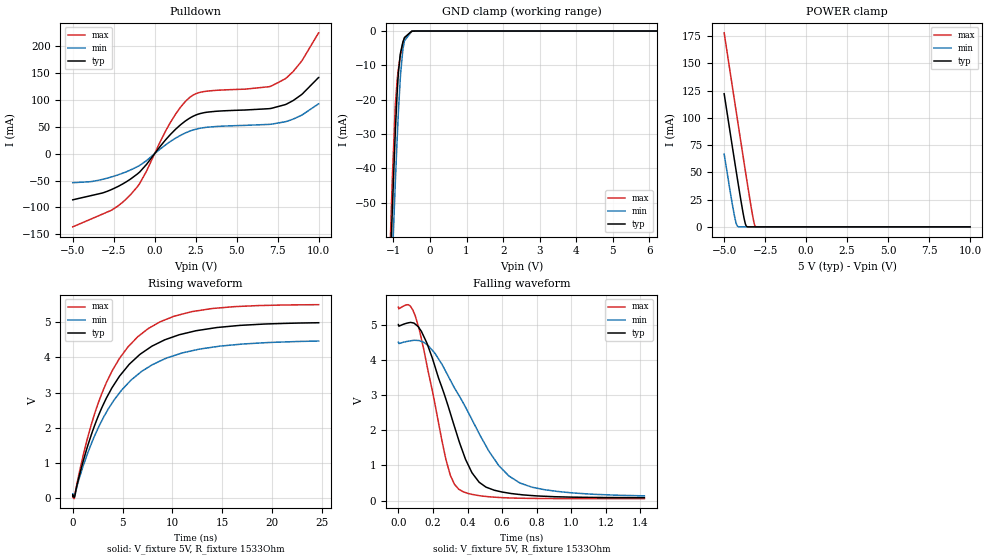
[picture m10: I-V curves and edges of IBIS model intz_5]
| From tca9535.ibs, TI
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|   intz_5 Model
[Model]   intz_5
Model_type   Open_sink
Polarity   Non-Inverting
Vmeas = 2.5
Vref = 5
Cref = 100pF
Rref = 1533
|   typ   min   max
|   (nom PVT)   (fast PVT)   (slow PVT)
C_comp   3.209e-12   3.204e-12   3.540e-12
| Where nom  PVT is Nominal Process, 5V, 27C
|   Fast PVT is Strong Process,  5.5V, -40C
|   Slow PVT is Weak Process,   4.5V, 100C
[Voltage Range]   5   4.5   5.5
|Junction Temperature
[Temperature Range]   27   100   -40
[Pullup Reference]   5   4.5   5.5
[Pulldown Reference]   0   0   0
[Power Clamp Reference]   5   4.5   5.5
[GND Clamp Reference]   0   0   0
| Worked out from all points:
|   slope of the pulldown table from 0 to 0.75 V, typ, clamps not added: 26.3 ohm
|   GND clamp passes 1 mA (typ) near -0.60 V on its own axis
|   POWER clamp passes 1 mA (typ) near -3.66 V on its own axis
|   falling waveform, V_fixture 5V, R_fixture 1533Ohm: 20-80 % time 201ps typ, 301ps min, 135ps max; typ from 5 V to 0.084 V
|   rising waveform, V_fixture 5V, R_fixture 1533Ohm: 20-80 % time 5.37ns typ, 5.74ns min, 4.93ns max; typ from 0.078 V to 4.98 V
[Pulldown]
|   Voltage   I(typ)   I(min)   I(max)
-5V       -85.83mA   -54.02mA   -136.1mA
-2.635V   -66.76mA   -43.31mA   -105.2mA
-1.486V   -47.45mA   -30.49mA   -76.69mA
-913.5mV  -33.98mA   -21.71mA   -55.33mA
967.5mV   36.03mA    22.95mA    58.62mA
2.117V    65.81mA    41.68mA    104.2mA
3.1V      76.74mA    48.82mA    116mA
7.101V    84.21mA    54.81mA    125.6mA
7.958V    91.23mA    59.35mA    139.2mA
8.447V    98.85mA    64.3mA     152.9mA
9.004V    111.1mA    72.36mA    174.1mA
10V       141.8mA    92.78mA    224.8mA
[GND Clamp]
|   Voltage   I(typ)   I(min)   I(max)
-5V       -1.737A    -1.579A    -1.998A
-1.085V   -68.6mA    -82.69mA   -60.63mA
-1.034V   -52.99mA   -67.79mA   -44mA
-1.03V    -51.64mA   -66.48mA   -42.61mA
-946.5mV  -28.53mA   -43.34mA   -21.14mA
-900.5mV  -18.27mA   -31.74mA   -14.42mA
-875mV    -13.78mA   -25.83mA   -11.89mA
-815mV    -6.977mA   -14.08mA   -7.383mA
-743mV    -3.229mA   -5.373mA   -3.548mA
-699mV    -1.904mA   -2.808mA   -1.974mA
-500mV    -56.39uA   -109.9uA   -29.75uA
10V       0A         0A         0A
[POWER Clamp]
|   Voltage   I(typ)   I(min)   I(max)
-5V       122.2mA    66.83mA    178.2mA
-4.519V   75.31mA    22.22mA    130.6mA
-4.343V   58.41mA    7.966mA    113.4mA
-4.235V   48.11mA    1.854mA    102.8mA
-4.15V    40.09mA    219.4uA    94.43mA
-3.865V   14.26mA    47.82nA    66.64mA
-3.71V    2.889mA    13.4nA     51.65mA
-3.61V    172.9uA    12.3nA     42.06mA
-3.272V   0A         0A         10.96mA
-3.163V   0A         0A         2.802mA
-3.091V   0A         0A         279.9uA
10V       0A         0A         0A
[Ramp]
R_load = 1533
|   typ   min   max
dV/dt_r   2.95311/5.42004e-09   2.63427/5.89243e-09   3.26857/4.94307e-09
dV/dt_f   2.95311/2.01074e-10   2.63427/3.0361e-10   3.26857/1.35007e-10
[Falling Waveform]
V_fixture = 5V
V_fixture_min = 4.5V
V_fixture_max = 5.5V
R_fixture = 1533Ohm
|   Time   V(typ)   V(min)   V(max)
0s        5V         4.5V       5.5V
55.06ps   5.047V     4.525V     5.564V
98.31ps   5.007V     4.552V     5.232V
164.6ps   4.475V     4.43V      3.847V
274.5ps   2.884V     3.662V     1.172V
349ps     1.717V     2.997V     323.2mV
467.2ps   521.7mV    1.905V     142.3mV
580.8ps   265.7mV    995.5mV    90.21mV
704.1ps   172.5mV    498.4mV    68.84mV
1.424ns   84.04mV    136.2mV    55.26mV
[Rising Waveform]
V_fixture = 5V
V_fixture_min = 4.5V
V_fixture_max = 5.5V
R_fixture = 1533Ohm
|   Time   V(typ)   V(min)   V(max)
0s        78.15mV    109.5mV    52.38mV
146.8ps   30.34mV    70.33mV    -11.89mV
1.414ns   1.409V     1.216V     1.636V
2.9ns     2.561V     2.195V     2.964V
4.687ns   3.464V     2.99V      3.97V
6.523ns   4.028V     3.512V     4.585V
8.771ns   4.433V     3.898V     5.01V
11.94ns   4.726V     4.185V     5.297V
16.74ns   4.906V     4.37V      5.445V
24.66ns   4.982V     4.462V     5.495V
